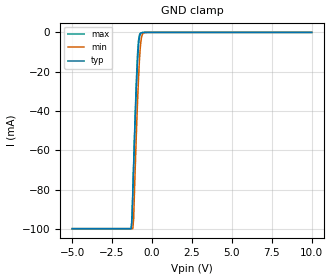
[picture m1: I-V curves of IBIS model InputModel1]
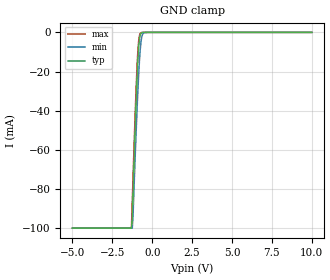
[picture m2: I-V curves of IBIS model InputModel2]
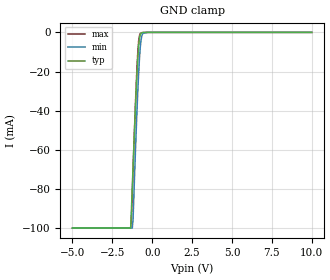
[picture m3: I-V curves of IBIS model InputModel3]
[IBIS Ver]   2.1
[File name]   e_800ce5.ibs   | e_= TSOP, f800ce= abbr chip name, 5= 5V Vcc
[File Rev]   2.00
[Date]   15-March-1996
[Source]   File generated from lab measurements at Intel Corporation
[Notes]   Rev 2.00 All data was replaced by actual measurements
   performed in a lab.
[Disclaimer] INTEL DEVELOPER'S SOFTWARE LICENSE AGREEMENT
| BY USING THIS SOFTWARE, YOU ARE AGREEING TO BE BOUND
| BY THE TERMS OF THIS AGREEMENT.  DO NOT USE THE SOFTWARE
| UNTIL YOU HAVE CAREFULLY READ AND AGREED TO THE FOLLOWING
| TERMS AND CONDITIONS.  IF YOU DO NOT AGREE TO THE TERMS
| OF THIS AGREEMENT, PROMPTLY RETURN THE SOFTWARE PACKAGE
| AND ANY ACCOMPANYING ITEMS.
| IF YOU USE THIS SOFTWARE, YOU WILL BE BOUND BY THE TERMS
| OF THIS AGREEMENT
| LICENSE: Intel Corporation ("Intel") grants you the non-exclusive right
| to use the enclosed software program ("Software").  You will not use,
| copy, modify, rent, sell or transfer the Software or any portion
| thereof, except as provided in this Agreement.
| System OEM Developers may:
| 1.   Copy the Software for support, backup or archival purposes;
| 2.   Install, use, or distribute Intel owned Software in object code
|   only;
| 3.   Modify and/or use Software source code that Intel directly makes
|   available to you as an OEM Developer;
| 4.   Install, use, modify, distribute, and/or make or have made
|   derivatives ("Derivatives") of Intel owned Software under the
|   terms and conditions in this Agreement, ONLY if you are a System
|   OEM Developer and NOT an end-user.
| RESTRICTIONS:
| YOU WILL NOT:
| 1.   Copy the Software, in whole or in part, except as provided for
|   in this Agreement;
| 2.   Decompile or reverse engineer any Software provided in object
|   code format;
| 3.   Distribute any Software or Derivative code to any end-users,
|   unless approved by Intel in a prior writing.
| TRANSFER: You may transfer the Software to another OEM
| Developer if the receiving party agrees to the terms of this
| Agreement at the sole risk of any receiving party.
| OWNERSHIP AND COPYRIGHT OF SOFTWARE:
| Title to the Software and all copies thereof remain with Intel
| or its vendors.  The Software is copyrighted and is protected by
| United States and international copyright laws.  You will not
| remove the copyright notice from the Software.  You agree to
| prevent any unauthorized copying of the Software.
| DERIVATIVE WORK: OEM Developers that make or have made
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[Copyright]   Copyright 1996, Intel Corporation, All Rights Reserved
[Component]   E28F800CE   | 48-lead TSOP package, 28F800CE
[Manufacturer]  Intel   | Boot Block (tm)
|   | operating in 5V Vcc range
[Package]
|Variable   typ   min   max
|The following values apply for the leadframe.
R_pkg   48.0m   41.0m   54.0m
L_pkg   4.92nH   4.44nH   5.39nH
C_pkg   0.48pF   0.45pF   0.50pF
|*****************************Pin Definitions**********************************
[Pin]   signal_name   model_name   R_pin   L_pin   C_pin
 1   A15   InputModel3
 2   A14   InputModel3
 3   A13   InputModel3
 4   A12   InputModel3
 5   A11   InputModel3
 6   A10   InputModel3
 7   A09   InputModel3
 8   A08   InputModel3
 9   NC   InputModel4
10   NC   InputModel4
11   WE#   InputModel1
12   RP#   InputModel1
13   VPP   POWER
14   WP#   InputModel1
15   NC   InputModel4
16   A18   InputModel3
17   A17   InputModel3
18   A07   InputModel3
19   A06   InputModel3
20   A05   InputModel3
21   A04   InputModel3
22   A03   InputModel3
23   A02   InputModel3
24   A01   InputModel3
25   A00   InputModel2
26   CE#   InputModel1
27   GND   GND
28   OE#   InputModel1
29   DQ0   InputOutput
30   DQ8   InputOutput
31   DQ1   InputOutput
32   DQ9   InputOutput
33   DQ2   InputOutput
34   DQ10   InputOutput
35   DQ3   InputOutput
36   DQ11   InputOutput
37   VCC   POWER
38   DQ4   InputOutput
39   DQ12   InputOutput
40   DQ5   InputOutput
41   DQ13   InputOutput
42   DQ6   InputOutput
43   DQ14   InputOutput
44   DQ7   InputOutput
45   DQ15   InputOutput
46   GND   GND
47   BYTE#   InputModel2
48   A16   InputModel2
|***********************Input Model 4******************************
[Model]   InputModel4
Model_type   Input
|   Model for NC pins (Numbers 9,10 & 15).
Vinl = 0.8V
Vinh = 2.0V
|Variable   Typ   Min   Max
C_comp   5.61p   NA   7.6p
[Voltage Range]   5.0V   4.5V   5.5V
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| Models and submodels in the file (5): InputModel1 (Input), InputModel2 (Input), InputModel3 (Input), InputModel4 (Input), InputOutput (I/O)
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|*********************Input Model 1************************************
[Model]   InputModel1
Model_type   Input
|   Model for WE#, WP#, RP#, OE# & CE#.
Vinl = 0.8V
Vinh = 2.0V
|Variable   Typ   Min   Max
C_comp   5.61p   NA   7.6p
[Voltage Range]   5.0V   4.5V   5.5V
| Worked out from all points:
|   GND clamp passes 1 mA (typ) near -0.74 V on its own axis
[GND_clamp]
|Voltage  I(typ)   I(min)   I(max)
-5V       -99.85mA   -99.85mA   -99.85mA
-1.3V     -99.85mA   -99.85mA   -99.85mA
-1.25V    -93.26mA   -99.85mA   -95.79mA
-1.2V     -80.3mA    -99.85mA   -81.5mA
-1.15V    -67.6mA    -94.88mA   -67.39mA
-1V       -32.49mA   -56.57mA   -29.26mA
-900mV    -13.7mA    -33.97mA   -10.19mA
-850mV    -7.324mA   -24.38mA   -4.514mA
-750mV    -1.17mA    -9.368mA   -570.4uA
-650mV    -196.9uA   -2.246mA   -163.7uA
-500mV    -19.68uA   -149.2uA   0A
10V       0A         0A         0A
[Power_clamp]
| Input buffer circuits of this product do not intrinsically
| require a [Power_clamp] definition.  This zero current
| [Power_clamp] table is provided for the compatibility with
| some IBIS parsers.
|Voltage  I(typ)   I(min)   I(max)
-5V       0A         0A         0A
0V        0A         0A         0A
5V        0A         0A         0A
10V       0A         0A         0A
|*********************Input Model 2******************************
[Model]   InputModel2
Model_type   Input
|   Model for A[0], A[16] & BYTE# pins.
Vinl = 0.8V
Vinh = 2.0V
|Variable   Typ   Min   Max
C_comp   5.61p   NA   7.6p
[Voltage Range]   5.0V   4.5V   5.5V
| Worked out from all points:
|   GND clamp passes 1 mA (typ) near -0.74 V on its own axis
[GND_clamp]
|Voltage  I(typ)   I(min)   I(max)
-5V       -99.85mA   -99.85mA   -99.85mA
-1.3V     -99.85mA   -99.85mA   -99.7mA
-1.25V    -95.1mA    -99.85mA   -86.57mA
-1.2V     -81.91mA   -93.12mA   -73.81mA
-1.05V    -44.51mA   -59.81mA   -37.94mA
-950mV    -22.91mA   -39.4mA    -17.7mA
-900mV    -14.12mA   -30.1mA    -9.812mA
-850mV    -7.485mA   -21.87mA   -4.492mA
-750mV    -1.181mA   -8.658mA   -581.8uA
-650mV    0A         -2.149mA   -166uA
-500mV    0A         -145.6uA   -18.8uA
10V       0A         0A         0A
[Power_clamp]
| Input buffer circuits of this product do not intrinsically
| require a [Power_clamp] definition.  This zero current
| [Power_clamp] table is provided for the compatibility with
| some IBIS parsers.
|Voltage  I(typ)   I(min)   I(max)
-5V       0A         0A         0A
0V        0A         0A         0A
5V        0A         0A         0A
10V       0A         0A         0A
|***********************Input Model 3******************************
[Model]   InputModel3
Model_type   Input
|   Model for A[15:1] & A[17:18].
Vinl = 0.8V
Vinh = 2.0V
|Variable   Typ   Min   Max
C_comp   5.61p   NA   7.6p
[Voltage Range]   5.0V   4.5V   5.5V
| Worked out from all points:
|   GND clamp passes 1 mA (typ) near -0.74 V on its own axis
[GND_clamp]
|Voltage  I(typ)   I(min)   I(max)
-5V       -99.85mA   -99.86mA   -99.85mA
-1.35V    -99.85mA   -99.86mA   -99.85mA
-1.3V     -90.17mA   -99.86mA   -94.83mA
-1.25V    -79.25mA   -99.86mA   -82.83mA
-1.2V     -68.58mA   -95.57mA   -70.38mA
-1.05V    -38.07mA   -60.6mA    -36.34mA
-950mV    -20.19mA   -39.21mA   -17.09mA
-850mV    -7.009mA   -21.02mA   -4.405mA
-750mV    -1.188mA   -7.828mA   -577.2uA
-600mV    -101.4uA   -746.5uA   -94.18uA
-250mV    0A         0A         0A
10V       0A         0A         0A
[Power_clamp]
| Input buffer circuits of this product do not intrinsically
| require a [Power_clamp] definition.  This zero current
| [Power_clamp] table is provided for the compatibility with
| some IBIS parsers.
|Voltage  I(typ)   I(min)   I(max)
-5V       0A         0A         0A
0V        0A         0A         0A
5V        0A         0A         0A
10V       0A         0A         0A
